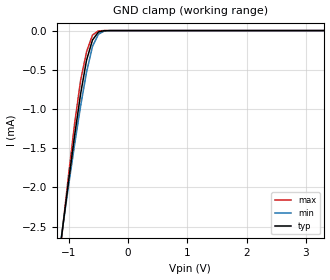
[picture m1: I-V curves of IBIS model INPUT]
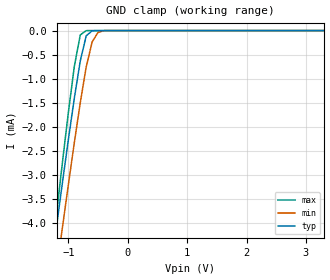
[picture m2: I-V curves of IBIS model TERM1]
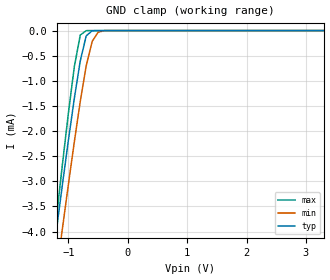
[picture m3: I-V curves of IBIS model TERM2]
|   PERICOM SEMICONDUCTOR CORP
|   IBIS Model of PI3USB14-A
|   Product Family: 3USB
|   TQFN (ZH) Package
[IBIS Ver] 3.2
[Comment char] |_char
[File Name] pi3usb14-a_zh_33v.ibs
[File Rev] 1.0
[Source] File originated at Pericom Semiconductor Corp.
[Date] 9/14/17
[Disclaimer] (C) Copyright PERICOM Semiconductor Corporation
   All rights reserved
  Pericom Semiconductor Corporation hereby grants the user of
  this IBIS model a non-exclusive, nontransferable license to
  use this IBIS model under the following terms.
  This IBIS model is provided on an "AS IS" basis and Pericom
  makes absolutely no warranty with respect to the information
  contained herein. PERICOM DISCLAIMS AND CUSTOMER WAIVES ALL
  WARRANTIES, EXPRESSED OR IMPLIED, INCLUDING WARRANTIES OF
  MERCHANTABILITY OR FITNESS FOR A PARTICULAR PURPOSE. The
  entire risk as to quality and performance is with the customer.
  Accordingly, in no event shall the company be liable for any
  damages, whether in contract or tort, including any lost
  profits or other incidental, consequential, exemplary, or
  punitive damages arising out of the use or application of the
  IBIS model provided in this package. Further, Pericom reserves
  the right to make changes without notice to any product herein
  to improve reliability, function, or design. Pericom does not
  convey any license under patent rights or any other intellectual
  property rights, including those of third parties.
  The user is granted this license only to use the IBIS model
  and is not granted rights to sell, load, rent, lease or license
  the IBIS model in whole or in part, or in modified form to anyone
  other than user. User may modify the IBIS model to suit its specific
  application but rights to derivative works and such modifications
  shall belong to Pericom.
  Pericom is not obligated to provide maintenance or support
  for the licensed IBIS model.
  Contact Pericom at ATTN: APPLICATION ENGINEERING / IBIS MODELS
  1545 Barber Lane Milpitas, CA 95035 USA.
[Component] PI3USB14-A
[Manufacturer] Pericom Semiconductor Corp.
[Package]
| variable   typ   min   max
R_pkg   0.02231ohm   NA   NA
L_pkg   0.85344nH   NA   NA
C_pkg   0.19700pF   NA   NA
[Pin]   signal_name   model_name   R_pin   L_pin   C_pin
1   NC   NC   0.02251 0.93000nH   0.23200pF
2   _EN   INPUT   0.02246 0.92500nH   0.22200pF
3   S1   INPUT   0.02231 0.85344nH   0.19700pF
4   IA3   TERM2   0.02215 0.78189nH   0.17200pF
5   IA2   TERM2   0.02201 0.71033nH   0.14700pF
6   IA1   TERM2   0.02201 0.71033nH   0.14700pF
7   IA0   TERM2   0.02215 0.78189nH   0.17200pF
8   YA   TERM1   0.02231 0.85344nH   0.19700pF
9   NC   NC   0.02246 0.92500nH   0.22200pF
10   GND   GND   0.02251 0.93000nH   0.23200pF
11   NC   NC   0.02251 0.93000nH   0.23200pF
12   YB   TERM1   0.02246 0.92500nH   0.22200pF
13   IB0   TERM2   0.02231 0.85344nH   0.19700pF
14   IB1   TERM2   0.02215 0.78189nH   0.17200pF
15   IB2   TERM2   0.02201 0.71033nH   0.14700pF
16   IB3   TERM2   0.02201 0.71033nH   0.14700pF
17   S0   INPUT   0.02215 0.78189nH   0.17200pF
18   NC   NC   0.02231 0.85344nH   0.19700pF
19   NC   NC   0.02246 0.92500nH   0.22200pF
20   VDD   POWER   0.02251 0.93000nH   0.23200pF
[Series Switch Groups]
On 0 /
Off 1 2 3 /
[Series Pin Mapping]   pin_2   model_name  function_table_group
4   8   SWITCH1   3   | S1-0 = 3
5   8   SWITCH1   2   | S1-0 = 2
6   8   SWITCH1   1   | S1-0 = 1
7   8   SWITCH1   0   | S1-0 = 0
13   12   SWITCH1   0   | S1-0 = 0
14   12   SWITCH1   1   | S1-0 = 1
15   12   SWITCH1   2   | S1-0 = 2
16   12   SWITCH1   3   | S1-0 = 3
|   Model SWITCH1
[Model] SWITCH1
Model_type Series_switch
| variable   typ   min   max
C_comp   7.70pF   7.60pF   7.80pF
[Voltage Range]   3.300V   2.970V   3.630V
[POWER Clamp Reference]   3.300V   2.970V   3.630V
[GND Clamp Reference]   0.000V   0.000V   0.000V
[On]
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[OFF]
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| Models and submodels in the file (4): INPUT (Input), SWITCH1 (Series_switch), TERM1 (Terminator), TERM2 (Terminator)
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|   Model INPUT
[Model] INPUT
Model_type Input
Vinl = 0.80V
Vinh = 2.00V
| variable   typ   min   max
C_comp   2.00pF   1.95pF   2.05pF
[Voltage Range]   3.300V   2.970V   3.630V
[POWER Clamp Reference]   3.300V   2.970V   3.630V
[GND Clamp Reference]   0.000V   0.000V   0.000V
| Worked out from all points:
|   GND clamp passes 1 mA (typ) near -0.84 V on its own axis
[GND Clamp]
| Voltage   I(typ)   I(min)   I(max)
-3.3V     -17.17mA   -15.62mA   -19.25mA
-1.2V     -3.11mA    -3.044mA   -3.202mA
-1.1V     -2.497mA   -2.495mA   -2.499mA
-1V       -1.901mA   -1.96mA    -1.819mA
-900mV    -1.331mA   -1.445mA   -1.178mA
-800mV    -805.5uA   -960.3uA   -633.7uA
-700mV    -377.2uA   -528.3uA   -270.1uA
-600mV    -120.6uA   -203uA     -57.04uA
-500mV    -17.99uA   -45.55uA   -3.824uA
-400mV    -1.285uA   -5.638uA   -103.3nA
-300mV    -57.05nA   -466.3nA   -1.677nA
3.3V      0A         232.8pA    174.6pA
[POWER Clamp]   |Note: Vtable = Vcc - Voutput
| Voltage   I(typ)   I(min)  I(max)
0V        0A         0A         0A
3.3V      0A         0A         0A
|   Model TERM1
[Model] TERM1
Model_type Terminator
| variable   typ   min   max
C_comp   4.40pF   4.35pF   4.45pF
[Voltage Range]   3.300V   2.970V   3.630V
[POWER Clamp Reference]   3.300V   2.970V   3.630V
[GND Clamp Reference]   0.000V   0.000V   0.000V
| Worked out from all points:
|   GND clamp passes 1 mA (typ) near -0.85 V on its own axis
[GND Clamp]
| Voltage   I(typ)   I(min)  I(max)
-3.3V     -24.26mA   -24.79mA   -27.56mA
-1.3V     -5.005mA   -5.913mA   -4.903mA
-1.2V     -4.075mA   -4.998mA   -3.81mA
-1.1V     -3.158mA   -4.091mA   -2.736mA
-1V       -2.263mA   -3.199mA   -1.698mA
-900mV    -1.405mA   -2.33mA    -743uA
-800mV    -631.7uA   -1.5mA     -90.43uA
-700mV    -108.7uA   -756.8uA   -982.7nA
-600mV    -4.457uA   -235.6uA   -7.749nA
-500mV    -277.3nA   -37.13uA   -225.6pA
-400mV    -6.032nA   -1.544uA   -109.1pA
3.3V      232.8pA    174.6pA    232.8pA
[POWER Clamp]   |Note: Vtable = Vcc - Voutput
| Voltage   I(typ)   I(min)  I(max)
0V        0A         0A         0A
3.3V      0A         0A         0A
|   Model TERM2
[Model] TERM2
Model_type Terminator
| variable   typ   min   max
C_comp   2.20pF   2.15pF   2.25pF
[Voltage Range]   3.300V   2.970V   3.630V
[POWER Clamp Reference]   3.300V   2.970V   3.630V
[GND Clamp Reference]   0.000V   0.000V   0.000V
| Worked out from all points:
|   GND clamp passes 1 mA (typ) near -0.85 V on its own axis
[GND Clamp]
| Voltage   I(typ)   I(min)  I(max)
-3.3V     -23.89mA   -24.35mA   -27.15mA
-1.3V     -4.873mA   -5.725mA   -4.783mA
-1.2V     -3.958mA   -4.824mA   -3.708mA
-1.1V     -3.058mA   -3.934mA   -2.655mA
-1V       -2.182mA   -3.061mA   -1.641mA
-900mV    -1.347mA   -2.212mA   -716.2uA
-800mV    -602.4uA   -1.409mA   -88.66uA
-700mV    -105.2uA   -700uA     -982.1nA
-600mV    -4.438uA   -217.2uA   -7.771nA
-500mV    -276.7nA   -33.56uA   -247.4pA
-400mV    -6.061nA   -1.497uA   -131pA
3.3V      174.6pA    174.6pA    116.4pA
[POWER Clamp]   |Note: Vtable = Vcc - Voutput
| Voltage   I(typ)   I(min)  I(max)
0V        0A         0A         0A
3.3V      0A         0A         0A
